{attribute 'qualified_only'}
VAR_GLOBAL
	HeartBeat:REAL;
//HW
	NDO:STR_NDO;
	AO:STR_AO;	
//Config
	PMConfig:ConfigPM;	
	Chiller:ConfigChiller;	
	InnerChiller:ConfigChiller;
	OuterChiller:ConfigChiller;
	TopChiller:ConfigChiller;	
	DryPump:ConfigDryPump;	
	Mfcgas1:ConfigMfcGas;
	MfcN2:ConfigMfcGas;
	MfcHe:ConfigMfcGas;	
	Pump:ConfigPump;	
	Purge:ConfigPurge;	
	PendulumHeater:ConfigHeater;
	LidHeater:ConfigHeater;
	ChamberHeater:ConfigHeater;
	ForelineHeater:ConfigHeater;
	STAGE:ConfigHeater;	
	PendulumValve:ConfigPendulumValve;		
//RECIPE
	Step_Num:INT;
	SetpArray:ARRAY[1..100] OF RecipeEachStep;	
//INTERLOCK
	TurboN2PurgePressure:INT;	//PS103		
//PROCESS
	Process_Start:BOOL;
	Process_Stop:BOOL;
	Warning_And_Alarm_RST:BOOL;	
END_VAR
